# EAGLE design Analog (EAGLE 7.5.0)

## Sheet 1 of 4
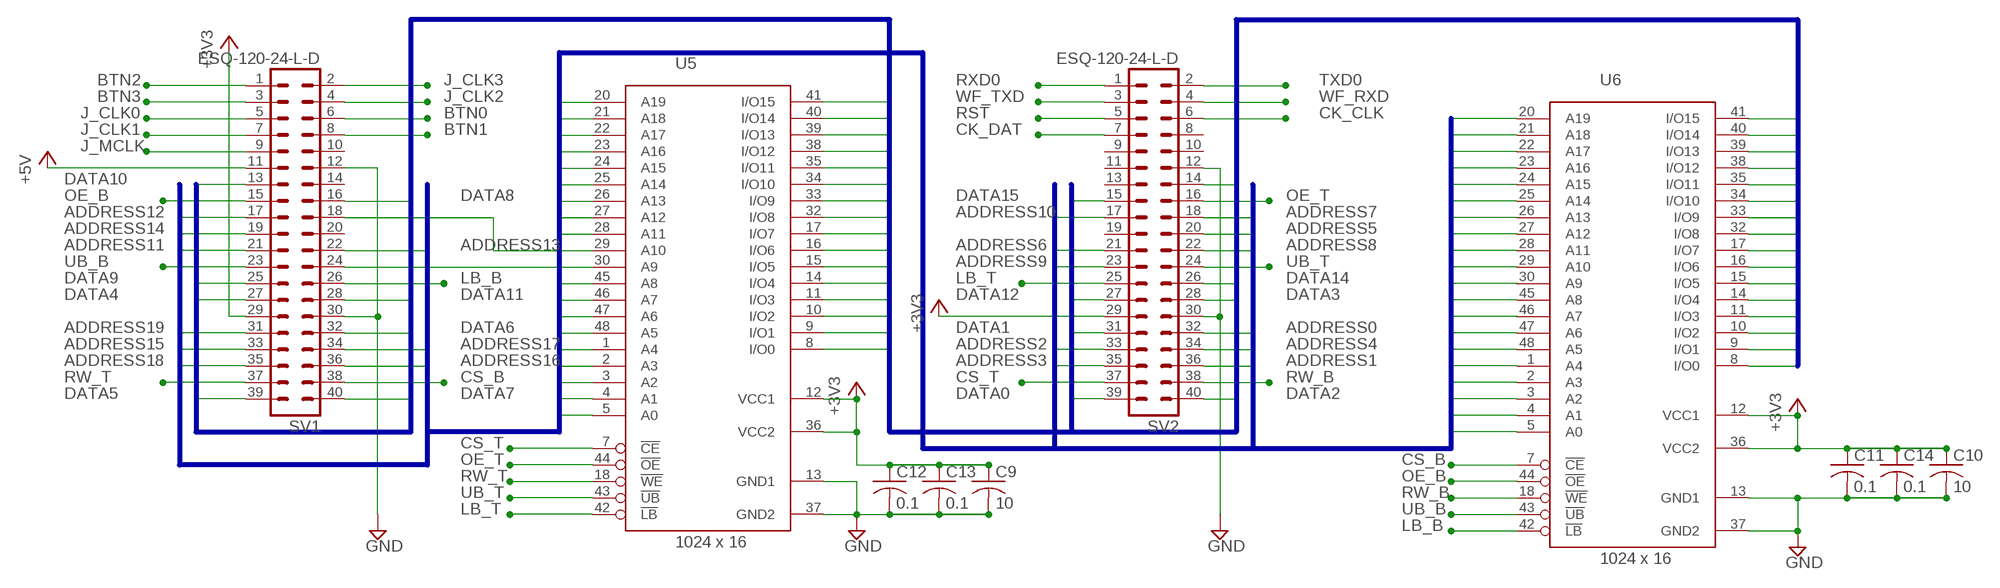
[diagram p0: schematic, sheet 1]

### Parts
C9  10  C-USC0805  [C0805]
C10  10  C-USC0805  [C0805]
C11  0.1  C-USC2012  [C2012]
C12  0.1  C-USC0805  [C0805]
C13  0.1  C-USC0805  [C0805]
C14  0.1  C-USC2012  [C2012]
SV1  ESQ-120-24-L-D  MA20-2  [MA20-2]
SV2  ESQ-120-24-L-D  MA20-2  [MA20-2]
U5  1024 x 16  IS62WV102416BLL-25T  [TSOP-I-48-12X40MM]
U6  1024 x 16  IS62WV102416BLL-25T  [TSOP-I-48-12X40MM]

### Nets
+3V3: C9.1 C10.1 C11.1 C12.1 C13.1 C14.1 SV1.29 SV2.29 U5.12(VCC1) U5.36(VCC2) U6.12(VCC1) U6.36(VCC2) ; also sheet 2,4
+5V: SV1.11 ; also sheet 3,4
ADDRESS0: SV2.32 U5.5(A0) U6.20(A19)
ADDRESS1: SV2.36 U5.4(A1) U6.21(A18)
ADDRESS2: SV2.33 U5.3(A2) U6.22(A17)
ADDRESS3: SV2.35 U5.2(A3) U6.23(A16)
ADDRESS4: SV2.34 U5.1(A4) U6.24(A15)
ADDRESS5: SV2.20 U5.48(A5) U6.25(A14)
ADDRESS6: SV2.21 U5.47(A6) U6.26(A13)
ADDRESS7: SV2.18 U5.46(A7) U6.27(A12)
ADDRESS8: SV2.22 U5.45(A8) U6.28(A11)
ADDRESS9: SV2.23 U6.30(A9)
ADDRESS9T: SV1.24 U5.30(A9)
ADDRESS10: SV2.17 U6.29(A10)
ADDRESS10T: SV1.18 U5.29(A10)
ADDRESS11: SV1.21 U5.28(A11) U6.45(A8)
ADDRESS12: SV1.17 U5.27(A12) U6.46(A7)
ADDRESS13: SV1.22 U5.26(A13) U6.47(A6)
ADDRESS14: SV1.19 U5.25(A14) U6.48(A5)
ADDRESS15: SV1.33 U5.24(A15) U6.1(A4)
ADDRESS16: SV1.36 U5.23(A16) U6.2(A3)
ADDRESS17: SV1.34 U5.22(A17) U6.3(A2)
ADDRESS18: SV1.35 U5.21(A18) U6.4(A1)
ADDRESS19: SV1.31 U5.20(A19) U6.5(A0)
BTN0: SV1.6 ; also sheet 3
BTN1: SV1.8 ; also sheet 3
BTN2: SV1.1 ; also sheet 3
BTN3: SV1.3 ; also sheet 3
CK_CLK: SV2.6 ; also sheet 4
CK_DAT: SV2.7 ; also sheet 4
CS_B: SV1.38 U6.7(!CE)
CS_T: SV2.37 U5.7(!CE)
DATA0: SV2.39 U5.8(I/O0) U6.17(I/O7)
DATA1: SV2.31 U5.9(I/O1) U6.16(I/O6)
DATA2: SV2.40 U5.10(I/O2) U6.15(I/O5)
DATA3: SV2.28 U5.11(I/O3) U6.14(I/O4)
DATA4: SV1.27 U5.14(I/O4) U6.11(I/O3)
DATA5: SV1.39 U5.15(I/O5) U6.10(I/O2)
DATA6: SV1.32 U5.16(I/O6) U6.9(I/O1)
DATA7: SV1.40 U5.17(I/O7) U6.8(I/O0)
DATA8: SV1.16 U5.32(I/O8) U6.41(I/O15)
DATA9: SV1.25 U5.33(I/O9) U6.40(I/O14)
DATA10: SV1.13 U5.34(I/O10) U6.39(I/O13)
DATA11: SV1.28 U5.35(I/O11) U6.38(I/O12)
DATA12: SV2.27 U5.38(I/O12) U6.35(I/O11)
DATA13: SV2.14 U5.39(I/O13) U6.34(I/O10)
DATA14: SV2.26 U5.40(I/O14) U6.33(I/O9)
DATA15: SV2.15 U5.41(I/O15) U6.32(I/O8)
GND: C9.2 C10.2 C11.2 C12.2 C13.2 C14.2 SV1.12 SV1.30 SV2.12 SV2.30 U5.13(GND1) U5.37(GND2) U6.13(GND1) U6.37(GND2) ; also sheet 2,3,4
J_CLK0: SV1.5 ; also sheet 3
J_CLK1: SV1.7 ; also sheet 3
J_CLK2: SV1.4 ; also sheet 3
J_CLK3: SV1.2 ; also sheet 3
J_MCLK: SV1.9 ; also sheet 3
LB_B: SV1.26 U6.42(!LB)
LB_T: SV2.25 U5.42(!LB)
OE_B: SV1.15 U6.44(!OE)
OE_T: SV2.16 U5.44(!OE)
RST: SV2.5 ; also sheet 4
RW_B: SV2.38 U6.18(!WE)
RW_T: SV1.37 U5.18(!WE)
RXD0: SV2.1 ; also sheet 2
TXD0: SV2.2 ; also sheet 2
UB_B: SV1.23 U6.43(!UB)
UB_T: SV2.24 U5.43(!UB)
WF_RXD: SV2.4 ; also sheet 4
WF_TXD: SV2.3 ; also sheet 4
Unconnected: SV1.10 SV1.14 SV1.20 SV2.8 SV2.9 SV2.10 SV2.11 SV2.13 SV2.19

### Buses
DATA[0..15]
ADDRESS[0..19]

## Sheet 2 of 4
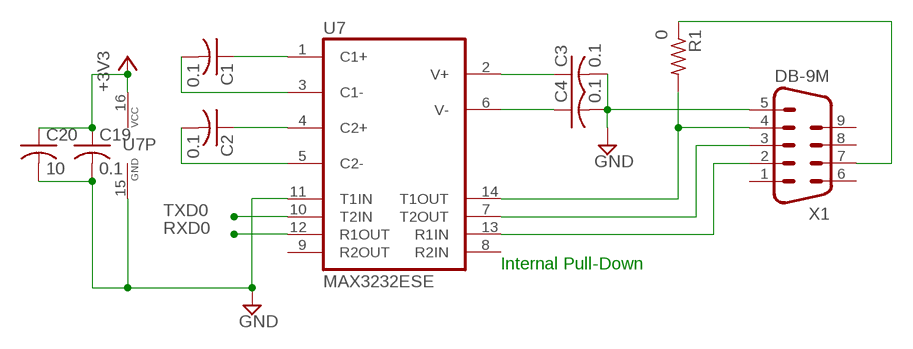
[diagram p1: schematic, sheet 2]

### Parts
C1  0.1  C-USC0805  [C0805]
C2  0.1  C-USC0805  [C0805]
C3  0.1  C-USC0805  [C0805]
C4  0.1  C-USC0805  [C0805]
C19  0.1  C-USC0805  [C0805]
C20  10  C-USC0805  [C0805]
R1  0  R-US_M0805  [M0805]
U7  MAX3232ESE  [SO16]
X1  DB-9M  M09HP  [M09HP]

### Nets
+3V3: C19.1 C20.1 U7.16(VCC) ; also sheet 1,4
GND: C3.2 C4.2 C19.2 C20.2 U7.11(T1IN) U7.15(GND) X1.5 ; also sheet 1,3,4
N$1: C1.1 U7.1(C1+)
N$2: C1.2 U7.3(C1-)
N$3: C2.1 U7.4(C2+)
N$4: C2.2 U7.5(C2-)
N$5: C3.1 U7.2(V+)
N$6: C4.1 U7.6(V-)
N$8: U7.13(R1IN) X1.2
N$9: U7.7(T2OUT) X1.3
N$27: R1.1 X1.7
N$28: R1.2 U7.14(T1OUT) X1.4
RXD0: U7.12(R1OUT) ; also sheet 1
TXD0: U7.10(T2IN) ; also sheet 1
Unconnected: U7.8(R2IN) U7.9(R2OUT) X1.1 X1.6 X1.8 X1.9

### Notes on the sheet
- Internal Pull-Down

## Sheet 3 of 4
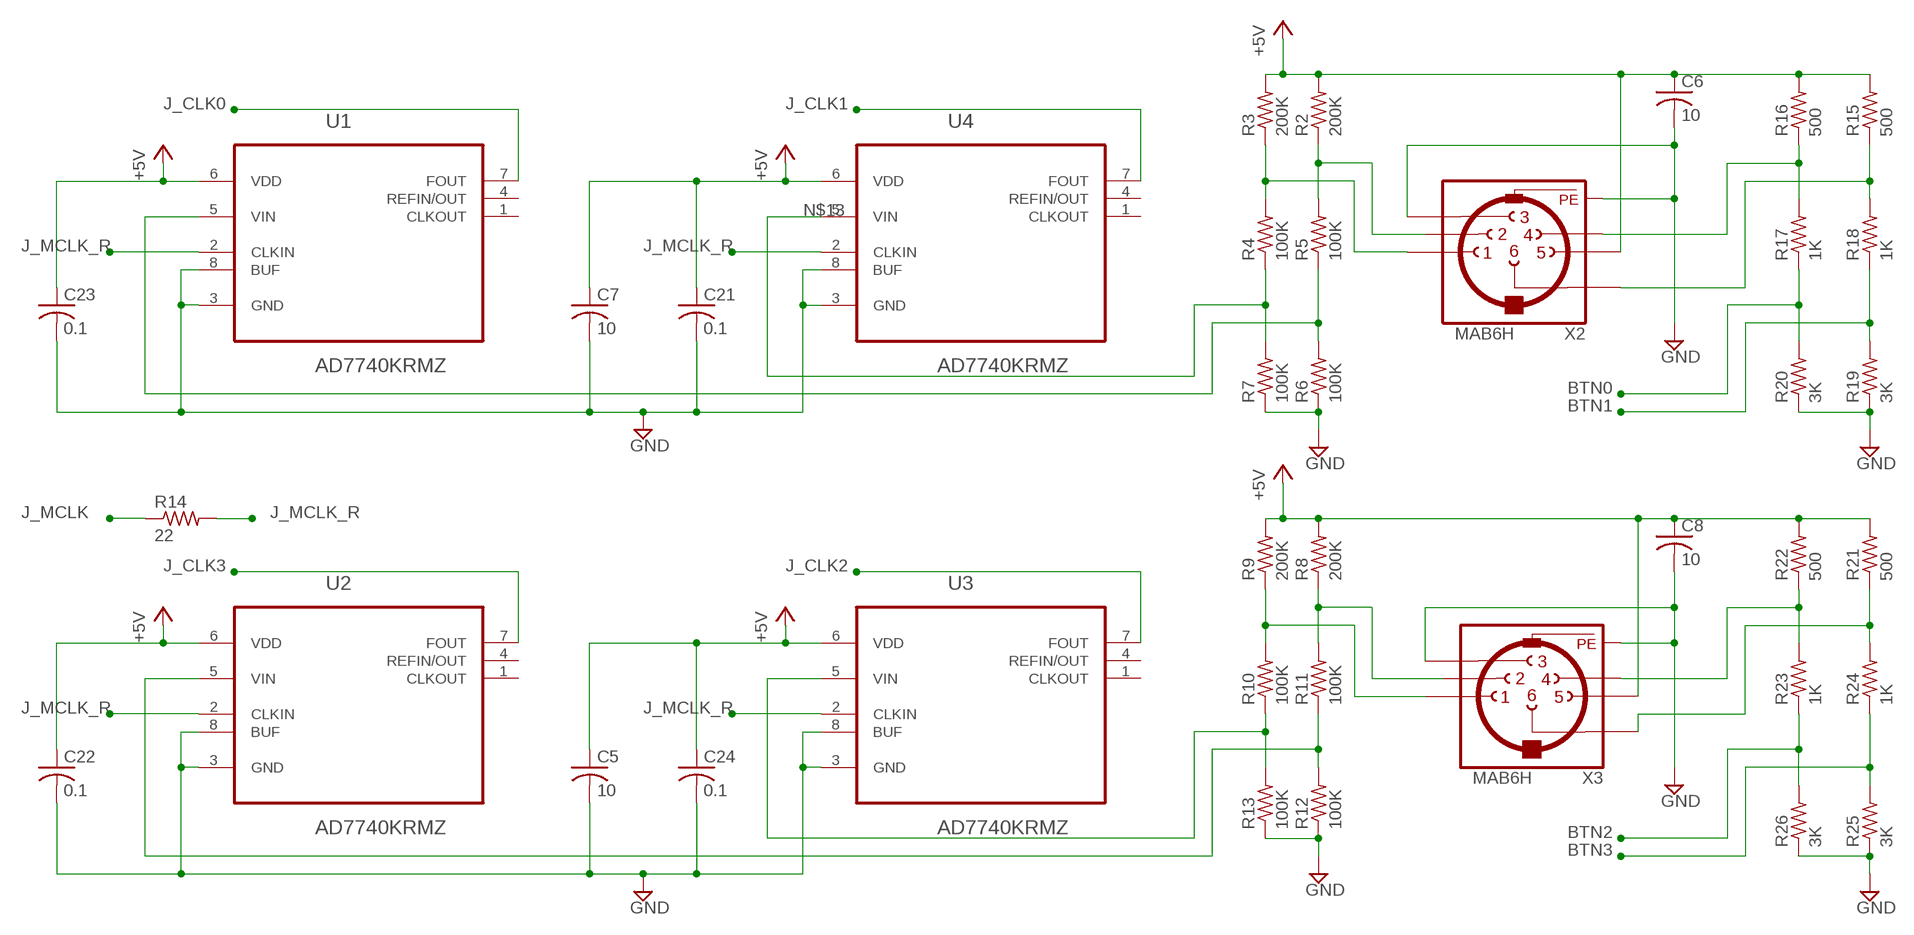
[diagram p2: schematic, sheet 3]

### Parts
C5  10  C-USC0805K  [C0805K]
C6  10  C-USC0805K  [C0805K]
C7  10  C-USC0805K  [C0805K]
C8  10  C-USC0805K  [C0805K]
C21  0.1  C-USC0805K  [C0805K]
C22  0.1  C-USC0805K  [C0805K]
C23  0.1  C-USC0805K  [C0805K]
C24  0.1  C-USC0805K  [C0805K]
R2  200K  R-US_M0805  [M0805]
R3  200K  R-US_M0805  [M0805]
R4  100K  R-US_M0805  [M0805]
R5  100K  R-US_M0805  [M0805]
R6  100K  R-US_M0805  [M0805]
R7  100K  R-US_M0805  [M0805]
R8  200K  R-US_M0805  [M0805]
R9  200K  R-US_M0805  [M0805]
R10  100K  R-US_M0805  [M0805]
R11  100K  R-US_M0805  [M0805]
R12  100K  R-US_M0805  [M0805]
R13  100K  R-US_M0805  [M0805]
R14  22  R-US_R0805  [R0805]
R15  500  R-US_R0805  [R0805]
R16  500  R-US_R0805  [R0805]
R17  1K  R-US_R0805  [R0805]
R18  1K  R-US_R0805  [R0805]
R19  3K  R-US_R0805  [R0805]
R20  3K  R-US_R0805  [R0805]
R21  500  R-US_R0805  [R0805]
R22  500  R-US_R0805  [R0805]
R23  1K  R-US_R0805  [R0805]
R24  1K  R-US_R0805  [R0805]
R25  3K  R-US_R0805  [R0805]
R26  3K  R-US_R0805  [R0805]
U1  AD7740KRMZ  [SOIC65P490X109-8N]
U2  AD7740KRMZ  [SOIC65P490X109-8N]
U3  AD7740KRMZ  [SOIC65P490X109-8N]
U4  AD7740KRMZ  [SOIC65P490X109-8N]
X2  MAB6H  [MAB6H]
X3  MAB6H  [MAB6H]

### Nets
+5V: C5.1 C6.1 C7.1 C8.1 C21.1 C22.1 C23.1 C24.1 R2.2 R3.2 R8.2 R9.2 R15.2 R16.2 R21.2 R22.2 U1.6(VDD) U2.6(VDD) U3.6(VDD) U4.6(VDD) X2.5 X3.5 ; also sheet 1,4
BTN0: R17.1 R20.2 ; also sheet 1
BTN1: R18.1 R19.2 ; also sheet 1
BTN2: R23.1 R26.2 ; also sheet 1
BTN3: R24.1 R25.2 ; also sheet 1
GND: C5.2 C6.2 C7.2 C8.2 C21.2 C22.2 C23.2 C24.2 R6.1 R7.1 R12.1 R13.1 R19.1 R20.1 R25.1 R26.1 U1.3(GND) U1.8(BUF) U2.3(GND) U2.8(BUF) U3.3(GND) U3.8(BUF) U4.3(GND) U4.8(BUF) X2.3 X2.PE X2.PE@(PE) X3.3 X3.PE X3.PE@(PE) ; also sheet 1,2,4
J_CLK0: U1.7(FOUT) ; also sheet 1
J_CLK1: U4.7(FOUT) ; also sheet 1
J_CLK2: U3.7(FOUT) ; also sheet 1
J_CLK3: U2.7(FOUT) ; also sheet 1
J_MCLK: R14.1 ; also sheet 1
J_MCLK_R: R14.2 U1.2(CLKIN) U2.2(CLKIN) U3.2(CLKIN) U4.2(CLKIN)
N$11: R22.1 R23.2 X3.4
N$12: R3.1 R4.2 X2.1
N$13: R4.1 R7.2 U4.5(VIN)
N$14: R5.1 R6.2 U1.5(VIN)
N$15: R2.1 R5.2 X2.2
N$16: R21.1 R24.2 X3.6
N$17: R9.1 R10.2 X3.1
N$18: R10.1 R13.2 U3.5(VIN)
N$19: R11.1 R12.2 U2.5(VIN)
N$20: R8.1 R11.2 X3.2
N$21: R16.1 R17.2 X2.4
N$22: R15.1 R18.2 X2.6
Unconnected: U1.1(CLKOUT) U1.4(REFIN/OUT) U2.1(CLKOUT) U2.4(REFIN/OUT) U3.1(CLKOUT) U3.4(REFIN/OUT) U4.1(CLKOUT) U4.4(REFIN/OUT)

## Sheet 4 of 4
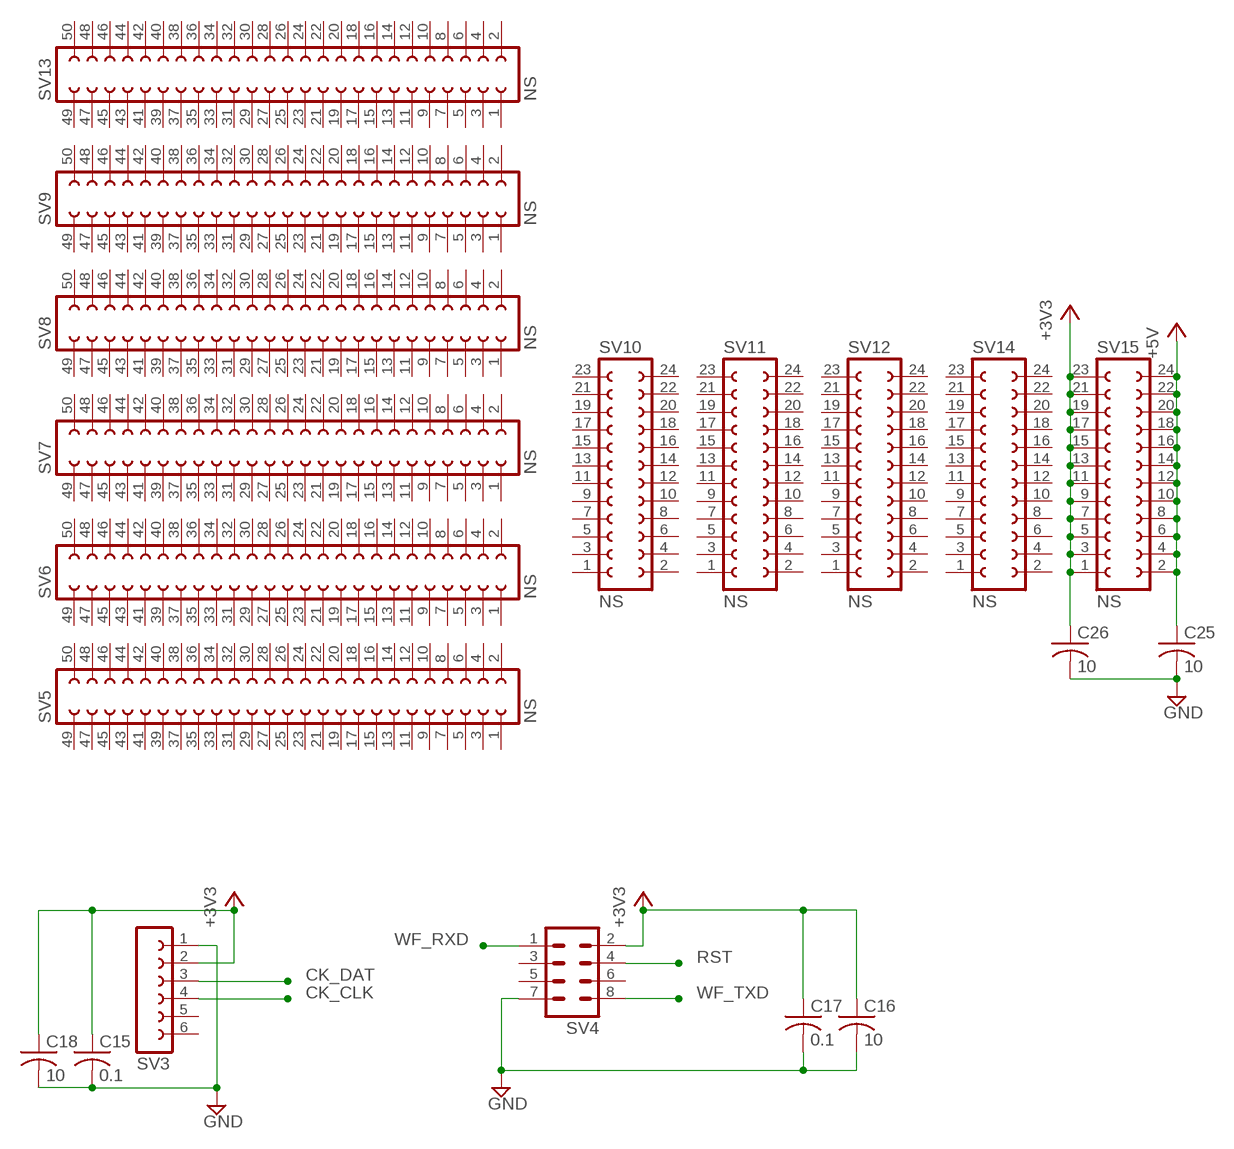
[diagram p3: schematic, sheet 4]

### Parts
C15  0.1  C-USC0805  [C0805]
C16  10  C-USC0805  [C0805]
C17  0.1  C-USC0805  [C0805]
C18  10  C-USC0805  [C0805]
C25  10  C-USC0805  [C0805]
C26  10  C-USC0805  [C0805]
SV3  FE06-1  [FE06]
SV4  MA04-2  [MA04-2]
SV5  NS  FE25-2  [FE25-2]
SV6  NS  FE25-2  [FE25-2]
SV7  NS  FE25-2  [FE25-2]
SV8  NS  FE25-2  [FE25-2]
SV9  NS  FE25-2  [FE25-2]
SV10  NS  FE12-2  [FE12-2]
SV11  NS  FE12-2  [FE12-2]
SV12  NS  FE12-2  [FE12-2]
SV13  NS  FE25-2  [FE25-2]
SV14  NS  FE12-2  [FE12-2]
SV15  NS  FE12-2  [FE12-2]

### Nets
+3V3: C15.1 C16.1 C17.1 C18.1 C26.1 SV3.2 SV4.2 SV15.1 SV15.3 SV15.5 SV15.7 SV15.9 SV15.11 SV15.13 SV15.15 SV15.17 SV15.19 SV15.21 SV15.23 ; also sheet 1,2
+5V: C25.1 SV15.2 SV15.4 SV15.6 SV15.8 SV15.10 SV15.12 SV15.14 SV15.16 SV15.18 SV15.20 SV15.22 SV15.24 ; also sheet 1,3
CK_CLK: SV3.4 ; also sheet 1
CK_DAT: SV3.3 ; also sheet 1
GND: C15.2 C16.2 C17.2 C18.2 C25.2 C26.2 SV3.1 SV4.7 ; also sheet 1,2,3
RST: SV4.4 ; also sheet 1
WF_RXD: SV4.1 ; also sheet 1
WF_TXD: SV4.8 ; also sheet 1
Unconnected: SV3.5 SV3.6 SV4.3 SV4.5 SV4.6 SV5.1 SV5.2 SV5.3 SV5.4 SV5.5 SV5.6 SV5.7 SV5.8 SV5.9 SV5.10 SV5.11 SV5.12 SV5.13 SV5.14 SV5.15 SV5.16 SV5.17 SV5.18 SV5.19 SV5.20 SV5.21 SV5.22 SV5.23 SV5.24 SV5.25 SV5.26 SV5.27 SV5.28 SV5.29 SV5.30 SV5.31 SV5.32 SV5.33 SV5.34 SV5.35 SV5.36 SV5.37 SV5.38 SV5.39 SV5.40 SV5.41 SV5.42 SV5.43 SV5.44 SV5.45 SV5.46 SV5.47 SV5.48 SV5.49 SV5.50 SV6.1 SV6.2 SV6.3 SV6.4 SV6.5 SV6.6 SV6.7 SV6.8 SV6.9 SV6.10 SV6.11 SV6.12 SV6.13 SV6.14 SV6.15 SV6.16 SV6.17 SV6.18 SV6.19 SV6.20 SV6.21 SV6.22 SV6.23 SV6.24 SV6.25 SV6.26 SV6.27 SV6.28 SV6.29 SV6.30 SV6.31 SV6.32 SV6.33 SV6.34 SV6.35 SV6.36 SV6.37 SV6.38 SV6.39 SV6.40 SV6.41 SV6.42 SV6.43 SV6.44 SV6.45 SV6.46 SV6.47 SV6.48 SV6.49 SV6.50 SV7.1 SV7.2 SV7.3 SV7.4 SV7.5 SV7.6 SV7.7 SV7.8 SV7.9 SV7.10 SV7.11 SV7.12 SV7.13 SV7.14 SV7.15 SV7.16 SV7.17 SV7.18 SV7.19 SV7.20 SV7.21 SV7.22 SV7.23 SV7.24 SV7.25 SV7.26 SV7.27 SV7.28 SV7.29 SV7.30 SV7.31 SV7.32 SV7.33 SV7.34 SV7.35 SV7.36 SV7.37 SV7.38 SV7.39 SV7.40 SV7.41 SV7.42 SV7.43 SV7.44 SV7.45 SV7.46 SV7.47 SV7.48 SV7.49 SV7.50 SV8.1 SV8.2 SV8.3 SV8.4 SV8.5 SV8.6 SV8.7 SV8.8 SV8.9 SV8.10 SV8.11 SV8.12 SV8.13 SV8.14 SV8.15 SV8.16 SV8.17 SV8.18 SV8.19 SV8.20 SV8.21 SV8.22 SV8.23 SV8.24 SV8.25 SV8.26 SV8.27 SV8.28 SV8.29 SV8.30 SV8.31 SV8.32 SV8.33 SV8.34 SV8.35 SV8.36 SV8.37 SV8.38 SV8.39 SV8.40 SV8.41 SV8.42 SV8.43 SV8.44 SV8.45 SV8.46 SV8.47 SV8.48 SV8.49 SV8.50 SV9.1 SV9.2 SV9.3 SV9.4 SV9.5 SV9.6 SV9.7 SV9.8 SV9.9 SV9.10 SV9.11 SV9.12 SV9.13 SV9.14 SV9.15 SV9.16 SV9.17 SV9.18 SV9.19 SV9.20 SV9.21 SV9.22 SV9.23 SV9.24 SV9.25 SV9.26 SV9.27 SV9.28 SV9.29 SV9.30 SV9.31 SV9.32 SV9.33 SV9.34 SV9.35 SV9.36 SV9.37 SV9.38 SV9.39 SV9.40 SV9.41 SV9.42 SV9.43 SV9.44 SV9.45 SV9.46 SV9.47 SV9.48 SV9.49 SV9.50 SV10.1 SV10.2 SV10.3 SV10.4 SV10.5 SV10.6 SV10.7 SV10.8 SV10.9 SV10.10 SV10.11 SV10.12 SV10.13 SV10.14 SV10.15 SV10.16 SV10.17 SV10.18 SV10.19 SV10.20 SV10.21 SV10.22 SV10.23 SV10.24 SV11.1 SV11.2 SV11.3 SV11.4 SV11.5 SV11.6 SV11.7 SV11.8 SV11.9 SV11.10 SV11.11 SV11.12 SV11.13 SV11.14 SV11.15 SV11.16 SV11.17 SV11.18 SV11.19 SV11.20 SV11.21 SV11.22 SV11.23 SV11.24 SV12.1 SV12.2 SV12.3 SV12.4 SV12.5 SV12.6 SV12.7 SV12.8 SV12.9 SV12.10 SV12.11 SV12.12 SV12.13 SV12.14 SV12.15 SV12.16 SV12.17 SV12.18 SV12.19 SV12.20 SV12.21 SV12.22 SV12.23 SV12.24 SV13.1 SV13.2 SV13.3 SV13.4 SV13.5 SV13.6 SV13.7 SV13.8 SV13.9 SV13.10 SV13.11 SV13.12 SV13.13 SV13.14 SV13.15 SV13.16 SV13.17 SV13.18 SV13.19 SV13.20 SV13.21 SV13.22 SV13.23 SV13.24 SV13.25 SV13.26 SV13.27 SV13.28 SV13.29 SV13.30 SV13.31 SV13.32 SV13.33 SV13.34 SV13.35 SV13.36 SV13.37 SV13.38 SV13.39 SV13.40 SV13.41 SV13.42 SV13.43 SV13.44 SV13.45 SV13.46 SV13.47 SV13.48 SV13.49 SV13.50 SV14.1 SV14.2 SV14.3 SV14.4 SV14.5 SV14.6 SV14.7 SV14.8 SV14.9 SV14.10 SV14.11 SV14.12 SV14.13 SV14.14 SV14.15 SV14.16 SV14.17 SV14.18 SV14.19 SV14.20 SV14.21 SV14.22 SV14.23 SV14.24

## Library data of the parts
C1-C26 = rcl:C-US: CAPACITOR, American symbol
R1-R26 = rcl:R-US_: RESISTOR, American symbol
SV1 SV2 = con-lstb:MA20-2: PIN HEADER; OC_FARNELL: unknown; OC_NEWARK: unknown
SV3 = con-lsta:FE06-1: FEMALE HEADER; OC_FARNELL: unknown; OC_NEWARK: unknown
SV4 = con-lstb:MA04-2: PIN HEADER; OC_FARNELL: unknown; OC_NEWARK: unknown
SV5-SV9 SV13 = Gary_LBR:FE25-2: FEMALE HEADER; OC_FARNELL: unknown; OC_NEWARK: unknown
SV10-SV12 SV14 SV15 = Gary_LBR:FE12-2: FEMALE HEADER; OC_FARNELL: unknown; OC_NEWARK: unknown
U1-U4 = Analog Devices_By_element14_Batch_1:AD7740KRMZ: 3 V/5 V Low Power, Synchronous Voltage-to-Frequency Converter; MPN: AD7740KRMZ; OC_FARNELL: 1661051; OC_NEWARK: 59K5406; PACKAGE: SOIC-8; SUPPLIER: Analog Devices
U5 U6 = Gary_LBR:IS62WV102416BLL-*: 1024k x 16 high- speed low power CMOS static RAM 25ns access time 3.6V power supply
U7 = maxim:MAX3232*: True RS-232 Transceivers 3.0V to 5.5V, Low-Power up to 1Mbps, Using Four 0.1µF External Capacitors Source: http://pdfserv.maxim-ic.com/en/ds/MAX3222-MAX3241.pdf; MF: MAXIM; MPN: MAX3232ESE; OC_FARNELL: 9725539; OC_NEWARK: 79C3880
X1 = con-subd:M09: SUB-D; OC_FARNELL: unknown; OC_NEWARK: unknown
X2 X3 = con-hirschmann:MAB6H: Female CONNECTOR 6 pins with shield, horizontal (DIN 45322); MF: FARNELL; MPN: MAB 6 H; OC_FARNELL: 809901; OC_NEWARK: 67C7887

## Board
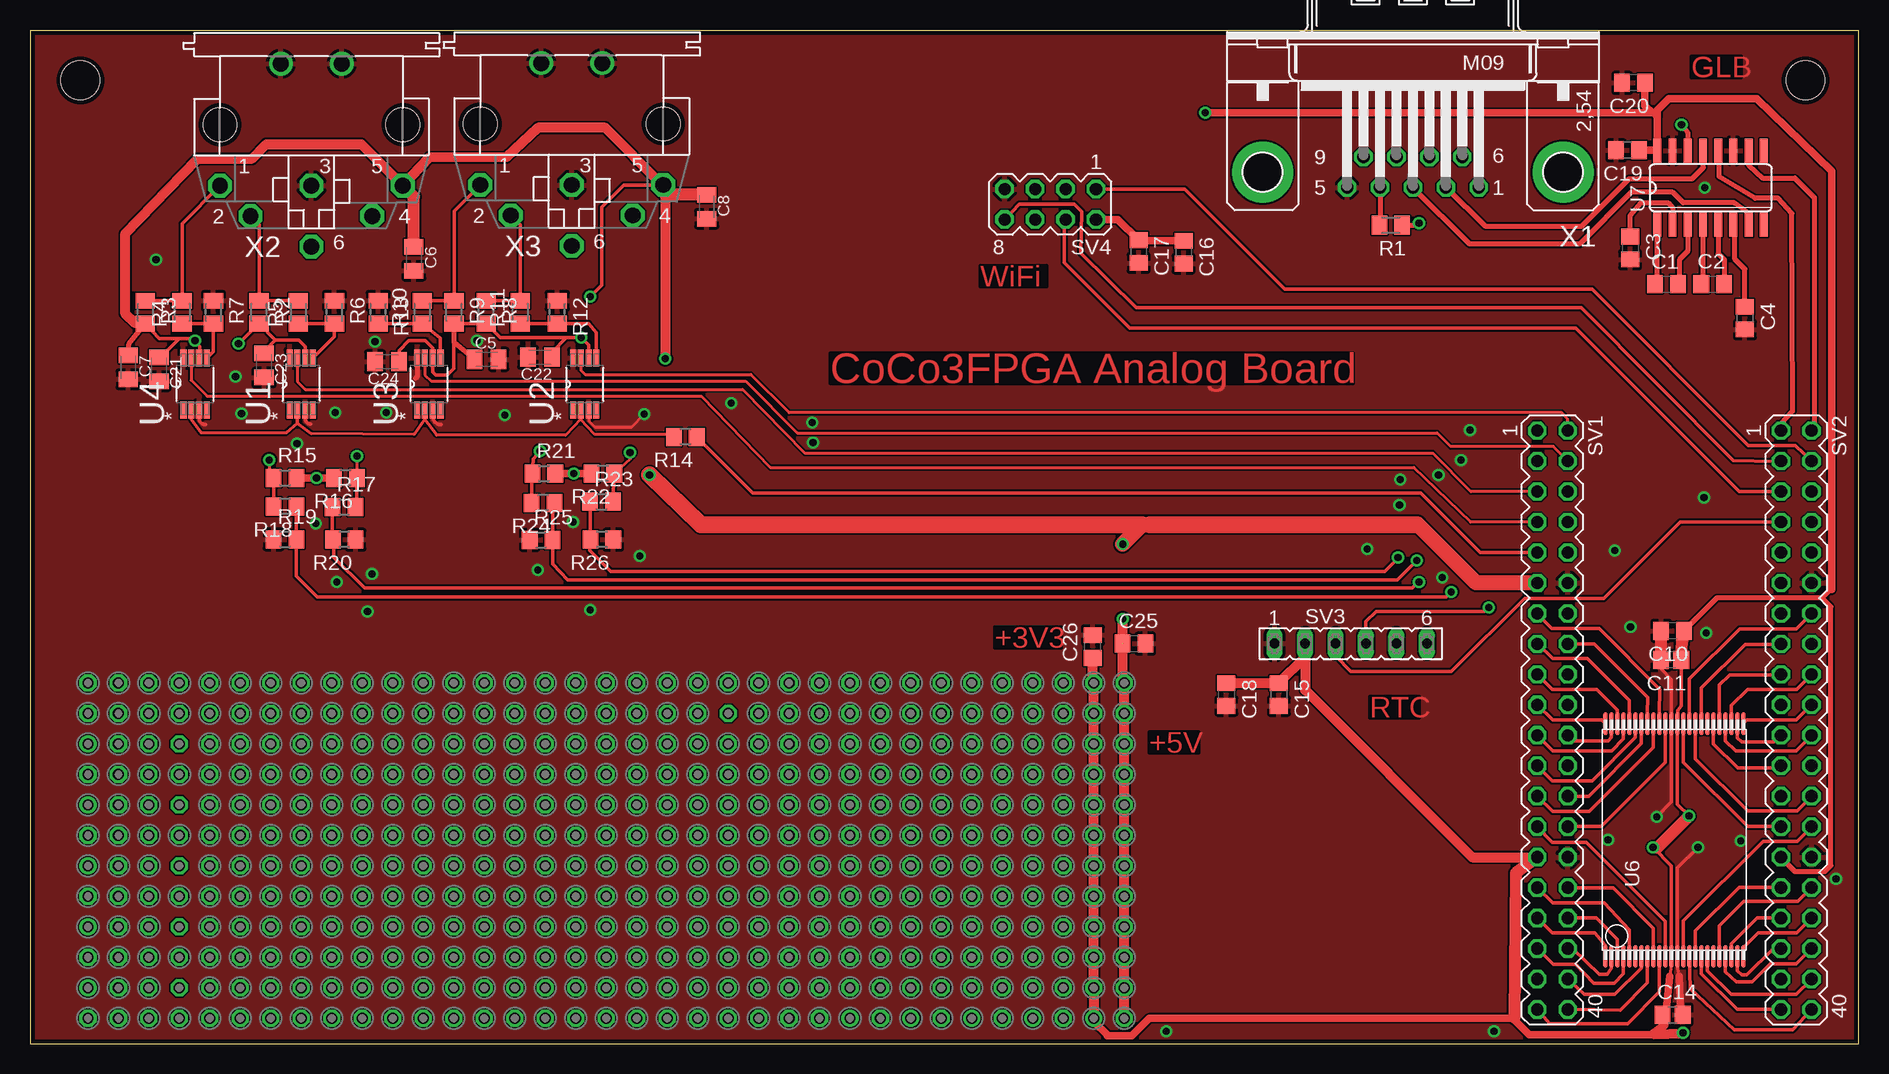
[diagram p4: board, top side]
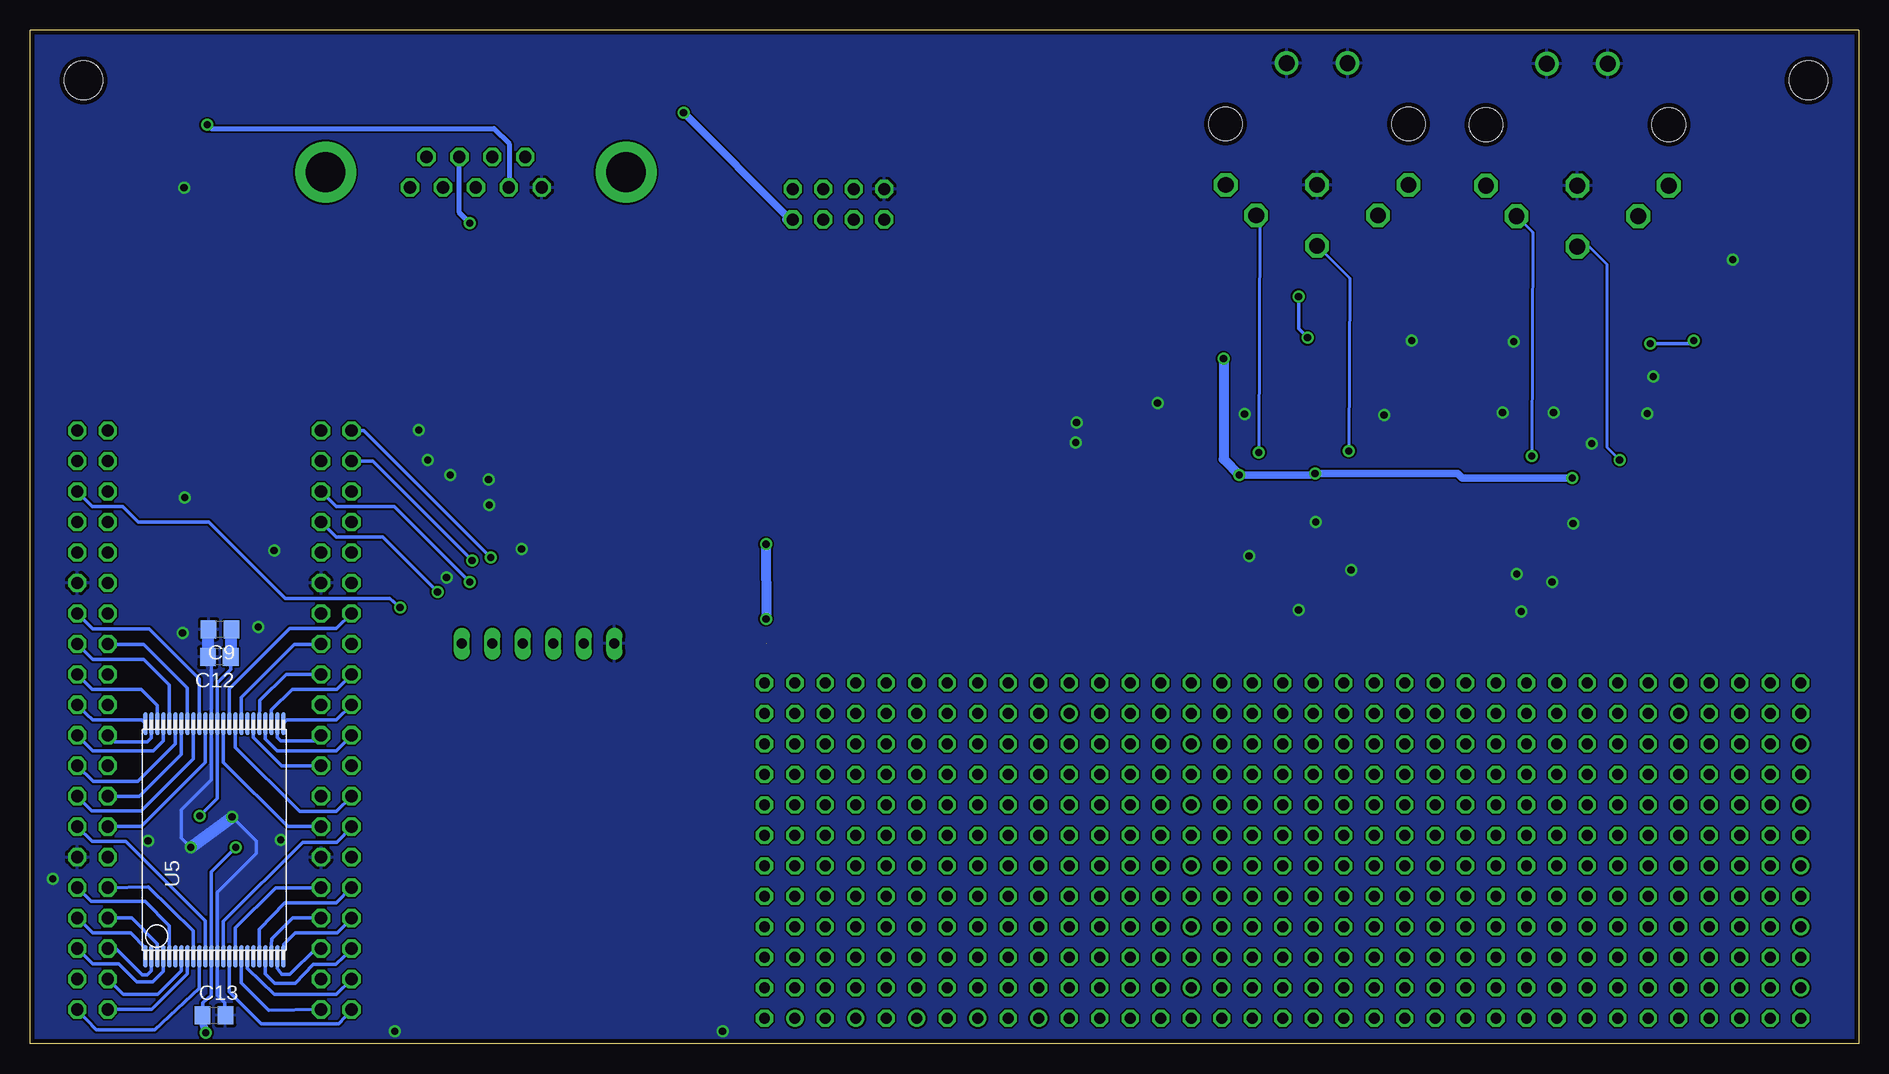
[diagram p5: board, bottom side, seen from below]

Size 152.4 x 84.53 mm. Coordinates in mm from the lower left corner, seen from the top.
Outline: 0,0 152.4,0 152.4,84.53 0,84.53 0,0
Copper layers (1*16): Top 0.035559375mm / dielectric 1.501140625mm / Bottom 0.035559375mm
Design rules "typical_4pcb": minimum track width 10mil, minimum drill 15mil, track to track 6mil, track to pad 6mil, pad to pad 6mil, via to via 6mil, smd to smd 6mil, copper to edge 15mil, drill to drill 8mil, minimum pad ring 10mil, minimum via ring 8mil, stop-mask expansion 4mil, vias tented up to drill 0mil, thermal gap 10mil
Holes 3.2 mm at 147.96,80.34 4.19,80.34

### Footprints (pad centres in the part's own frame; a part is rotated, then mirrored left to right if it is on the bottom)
C0805 = smd 1.3 x 1.5: 1 -0.95,0; 2 0.95,0
C0805K = smd 1.3 x 1.6: 1 -1,0; 2 1,0
C2012 = smd 1.3 x 1.5: 1 -0.85,0; 2 0.85,0
M0805 = smd 1.3 x 1.6: 1 -0.95,0; 2 0.95,0
R0805 = smd 1.3 x 1.5: 1 -0.95,0; 2 0.95,0
MA20-2 = drill 1.016 octagon: 1 -24.13,-1.27; 2 -24.13,1.27; 3 -21.59,-1.27; 4 -21.59,1.27; 5 -19.05,-1.27; 6 -19.05,1.27; 7 -16.51,-1.27; 8 -16.51,1.27; 9 -13.97,-1.27; 10 -13.97,1.27; 11 -11.43,-1.27; 12 -11.43,1.27; 13 -8.89,-1.27; 14 -8.89,1.27; 15 -6.35,-1.27; 16 -6.35,1.27; 17 -3.81,-1.27; 18 -3.81,1.27; 19 -1.27,-1.27; 20 -1.27,1.27; 21 1.27,-1.27; 22 1.27,1.27; 23 3.81,-1.27; 24 3.81,1.27; 25 6.35,-1.27; 26 6.35,1.27; 27 8.89,-1.27; 28 8.89,1.27; 29 11.43,-1.27; 30 11.43,1.27; 31 13.97,-1.27; 32 13.97,1.27; 33 16.51,-1.27; 34 16.51,1.27; 35 19.05,-1.27; 36 19.05,1.27; 37 21.59,-1.27; 38 21.59,1.27; 39 24.13,-1.27; 40 24.13,1.27
FE06 = drill 0.813 long: 1 -6.35,0; 2 -3.81,0; 3 -1.27,0; 4 1.27,0; 5 3.81,0; 6 6.35,0
MA04-2 = drill 1.016 octagon: 1 -3.81,-1.27; 2 -3.81,1.27; 3 -1.27,-1.27; 4 -1.27,1.27; 5 1.27,-1.27; 6 1.27,1.27; 7 3.81,-1.27; 8 3.81,1.27
FE25-2 = drill 0.914: 1 -30.48,1.27; 41 20.32,1.27 | drill 0.914 octagon: 2 -30.48,-1.27; 3 -27.94,1.27; 4 -27.94,-1.27; 5 -25.4,1.27; 6 -25.4,-1.27; 7 -22.86,1.27; 8 -22.86,-1.27; 9 -20.32,1.27; 10 -20.32,-1.27; 11 -17.78,1.27; 12 -17.78,-1.27; 13 -15.24,1.27; 14 -15.24,-1.27; 15 -12.7,1.27; 16 -12.7,-1.27; 17 -10.16,1.27; 18 -10.16,-1.27; 19 -7.62,1.27; 20 -7.62,-1.27; 21 -5.08,1.27; 22 -5.08,-1.27; 23 -2.54,1.27; 24 -2.54,-1.27; 25 0,1.27; 26 0,-1.27; 27 2.54,1.27; 28 2.54,-1.27; 29 5.08,1.27; 30 5.08,-1.27; 31 7.62,1.27; 32 7.62,-1.27; 33 10.16,1.27; 34 10.16,-1.27; 35 12.7,1.27; 36 12.7,-1.27; 37 15.24,1.27; 38 15.24,-1.27; 39 17.78,1.27; 40 17.78,-1.27; 42 20.32,-1.27; 43 22.86,1.27; 44 22.86,-1.27; 45 25.4,1.27; 46 25.4,-1.27; 47 27.94,1.27; 48 27.94,-1.27; 49 30.48,1.27; 50 30.48,-1.27
FE12-2 = drill 0.914: 1 -13.97,1.27 | drill 0.914 octagon: 2 -13.97,-1.27; 3 -11.43,1.27; 4 -11.43,-1.27; 5 -8.89,1.27; 6 -8.89,-1.27; 7 -6.35,1.27; 8 -6.35,-1.27; 9 -3.81,1.27; 10 -3.81,-1.27; 11 -1.27,1.27; 12 -1.27,-1.27; 13 1.27,1.27; 14 1.27,-1.27; 15 3.81,1.27; 16 3.81,-1.27; 17 6.35,1.27; 18 6.35,-1.27; 19 8.89,1.27; 20 8.89,-1.27; 21 11.43,1.27; 22 11.43,-1.27; 23 13.97,1.27; 24 13.97,-1.27
SOIC65P490X109-8N = smd 1.422 x 0.508: 1 -2.159,0.965; 2 -2.159,0.33; 3 -2.159,-0.33; 4 -2.159,-0.965; 5 2.159,-0.965; 6 2.159,-0.33; 7 2.159,0.33; 8 2.159,0.965
TSOP-I-48-12X40MM = smd 1.9 x 0.34: 1 -9.7,5.75; 2 -9.7,5.25; 3 -9.7,4.75; 4 -9.7,4.25; 5 -9.7,3.75; 6 -9.7,3.25; 7 -9.7,2.75; 8 -9.7,2.25; 9 -9.7,1.75; 10 -9.7,1.25; 11 -9.7,0.75; 12 -9.7,0.25; 13 -9.7,-0.25; 14 -9.7,-0.75; 15 -9.7,-1.25; 16 -9.7,-1.75; 17 -9.7,-2.25; 18 -9.7,-2.75; 19 -9.7,-3.25; 20 -9.7,-3.75; 21 -9.7,-4.25; 22 -9.7,-4.75; 23 -9.7,-5.25; 24 -9.7,-5.75; 25 9.7,-5.75; 26 9.7,-5.25; 27 9.7,-4.75; 28 9.7,-4.25; 29 9.7,-3.75; 30 9.7,-3.25; 31 9.7,-2.75; 32 9.7,-2.25; 33 9.7,-1.75; 34 9.7,-1.25; 35 9.7,-0.75; 36 9.7,-0.25; 37 9.7,0.25; 38 9.7,0.75; 39 9.7,1.25; 40 9.7,1.75; 41 9.7,2.25; 42 9.7,2.75; 43 9.7,3.25; 44 9.7,3.75; 45 9.7,4.25; 46 9.7,4.75; 47 9.7,5.25; 48 9.7,5.75
SO16 = smd 0.66 x 2.032: 1 -4.445,-3.073; 2 -3.175,-3.073; 3 -1.905,-3.073; 4 -0.635,-3.073; 5 0.635,-3.073; 6 1.905,-3.073; 7 3.175,-3.073; 8 4.445,-3.073; 9 4.445,3.073; 10 3.175,3.073; 11 1.905,3.073; 12 0.635,3.073; 13 -0.635,3.073; 14 -1.905,3.073; 15 -3.175,3.073; 16 -4.445,3.073
M09HP = drill 1.016 octagon: 1 -5.486,1.27; 2 -2.743,1.27; 3 0,1.27; 4 2.743,1.27; 5 5.486,1.27; 6 -4.115,-1.27; 7 -1.372,-1.27; 8 1.372,-1.27; 9 4.115,-1.27 | drill 3.302 pad 5.08: G1 -12.522,0; G2 12.522,0
MAB6H = drill 1.321 octagon: 1 7.62,5.08; 2 5.08,7.62; 3 0,5.08; 4 -5.08,7.62; 5 -7.62,5.08; 6 0,10.16 | drill 1.321: PE -2.54,-5.08; PE@ 2.54,-5.08 | hole 2.794: 7.62,0; -7.62,0

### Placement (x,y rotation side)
C1  136.37,63.34 0 top
C2  140.22,63.35 0 top
C3  133.35,66.35 270 top
C4  142.91,60.51 270 top
C5  38.06,57.07 0 top
C6  31.99,65.46 270 top
C7  8.19,56.41 270 top
C8  56.4,69.8 270 top
C9  136.56,34.56 180 bottom
C10  136.88,34.44 180 top
C11  136.75,32 180 top
C12  136.62,32.25 180 bottom
C13  137.06,2.38 0 bottom
C14  136.88,2.44 0 top
C15  104.06,29.12 270 top
C16  96.12,66 270 top
C17  92.38,66.06 270 top
C18  99.69,29.12 270 top
C19  133.12,74.5 180 top
C20  133.62,80.12 180 top
C21  10.75,56.25 270 top
C22  42.5,57.25 180 top
C23  19.5,56.56 270 top
C24  29.75,56.88 180 top
C25  92,33.38 0 top
C26  88.56,33.12 90 top
R1  113.39,68.25 180 top
R2  19.09,61 270 top
R3  9.62,61 270 top
R4  12.67,61 90 top
R5  22.35,61 90 top
R6  25.37,61 270 top
R7  15.29,61 270 top
R8  38.02,61 270 top
R9  35.34,61 270 top
R10  32.67,61 90 top
R11  40.84,61 90 top
R12  43.94,61 270 top
R13  29.01,61 270 top
R14  54.61,50.61 180 top
R15  21.24,47.19 0 top
R16  26.3,47.19 180 top
R17  26.17,44.77 0 top
R18  21.25,44.8 180 top
R19  21.25,42.07 0 top
R20  26.19,42.04 180 top
R21  42.82,47.56 0 top
R22  47.74,47.56 180 top
R23  47.63,45.2 0 top
R24  42.76,45.11 180 top
R25  42.59,42.02 0 top
R26  47.65,42.04 180 top
SV1  126.87,27 270 top
SV2  147.19,27 270 top
SV3  110.06,33.38 0 top
SV4  85.03,70 180 top
SV5  35.31,28.81 180 top
SV6  35.31,23.73 0 top
SV7  35.31,18.65 0 top
SV8  35.31,13.57 0 top
SV9  35.31,8.49 0 top
SV10  69.6,16.11 90 top
SV11  74.68,16.11 90 top
SV12  79.76,16.11 90 top
SV13  35.31,3.41 0 top
SV14  84.84,16.11 90 top
SV15  89.92,16.11 90 top
U1  22.6,55 90 top
U2  46.23,55 90 top
U3  33.24,55 90 top
U4  13.76,55 90 top
U5  137.03,17 90 bottom
U6  137.03,17 90 top
U7  140.05,71.38 0 top
X1  115.25,72.67 180 top
X2  23.45,76.63 180 top
X3  45.15,76.69 180 top

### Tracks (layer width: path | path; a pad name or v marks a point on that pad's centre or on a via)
+3V3  (via drill 0.6)
  Top 0.254: 137.31,27.55 U6.36 | 136.62,5.62 136.75,6.25 U6.12 | 123.56,2.12 123.62,2.12 123.69,2.12 123.69,2.19
  Top 0.305: C11.1 137.6,28.16 137.31,27.81 137.31,27.55 | v138.25,19 137.28,19.97 U6.36 | U6.12 136.78,14.84 v135.25,16.38
  Top 0.406: C14.1 136.12,2.44 136.31,2.44 | SV2.29 145.92,15.51 147.06,14.38 149.56,14.38 150.06,14.88 150.06,36.44 149.31,37.19 | 149.31,37.19 140.57,37.19 C10.1 | 150.12,37.88 150,37.88 149.31,37.19
  Top 0.61: SV4.2 90.66,68.73 C17.1 92.44,66.95 C16.1 | 136.31,2.44 136.62,5.62 | 135.06,0.75 136.12,1.56 | 135.06,0.75 135.31,0.81 | 150.12,37.88 150.12,72.75 143.88,78.81 136.56,78.81 135.6,77.86 135.6,77.31 | 135.6,77.31 U7.16 135.56,74.5 C19.1 | v97.94,77.62 135.19,77.62 | 135.19,77.62 135.29,77.62 135.6,77.31 | C20.1 134.57,78.24 135.19,77.62 | 135.06,0.75 124.94,0.75 123.56,2.12 | SV15.1 88.65,1.85 89.75,0.75 89.75,0.69 91.81,0.69 93.25,2.12 123.62,2.12
  Top 0.813: 136.12,1.56 136.12,2.44 | 135.31,0.81 137.81,0.88 | SV1.29 120.18,15.57 106.25,29.5 SV3.2 106.25,32.27 C15.1 C18.1 | SV15.1 SV15.3 SV15.5 SV15.7 SV15.9 SV15.11 SV15.13 SV15.15 SV15.17 SV15.19 SV15.21 SV15.23 88.58,30.16 C26.1
  Top 1.016: C11.1 arc-10 C10.1 | SV1.29 123.81,14.25 123.69,2.19 | v135.25,16.38 135.62,16.38 v138.25,19
  Bottom 0.305: v138.25,19 136.78,20.47 U5.36 136.78,30.09 135.68,31.2 C12.1 | v135.25,16.38 137.28,14.34 U5.12 137.28,6.43 137.31,4.06 138.01,3.42 C13.1
  Bottom 0.61: C13.1 138.01,1.76 137.93,1.51 v137.75,0.94 | 89.42,68.73 SV4.2 89.04,68.73 v97.94,77.62
  Bottom 0.813: C9.1 135.68,34.5
  Bottom 1.016: 135.68,34.5 C12.1
+5V  (via drill 0.6)  (1 unrouted)
  Top 0.305: R3.2 10.79,58.81 12.44,58.81 | U1.6 22.93,58.13 22.38,58.69 20.45,58.69 | 20.45,58.69 R2.2 19.05,60.05 v17.38,58.38 | U2.6 46.56,58.25 v45.94,58.88 44.69,58.88 | 44.69,58.88 39.2,58.88 R8.2 R9.2 35.31,60.02 35.31,56.31 34.75,55.75 33.81,55.75 33.56,56 33.56,56.06 33.57,56.07 U3.6 33.56,58 32.94,58.62 31.56,58.62 30.75,57.81 C24.1 | U4.6 14.12,57.2 14.12,58.12 v13.75,58.62 13.56,58.81 12.44,58.81 | X3.5 49.49,71.61 47.62,69.75 47.62,63.25 v46.69,62.31 | C21.1 10.88,57.25 12.44,58.81 | C23.1 19.5,57.73 20.45,58.69 | C22.1 43.5,57.69 44.69,58.88
  Top 0.406: C5.1 35.34,58.47 R9.2 | C7.1 8.24,58.34 R3.2
  Top 0.61: R21.2 v45.31,47.56 R22.2 | R16.2 v23.88,47.19 R15.2 | R3.2 8.76,60.11
  Top 0.813: v52.94,57.12 52.95,70.42 X3.5 52.7,71.61 47.94,76.38 42.31,76.38 39.69,73.94 33.27,73.88 X2.5 27.62,75 19.69,75 18.5,73.81 13.94,73.75 7.94,67.56 7.94,60.88 8.76,60.11 | 91.06,33.39 v91.06,35.44 | 91.19,33.23 C25.1 91.05,30.23 SV15.24 SV15.22 SV15.20 SV15.18 SV15.16 SV15.14 SV15.12 SV15.10 SV15.8 SV15.6 SV15.4 SV15.2
  Top 1.016: C6.1 31.99,70.63 X2.5 | C8.1 53.58,70.8 X3.5
  Top 1.27: SV1.11 120.51,38.43 115.62,43.31 115.6,43.29 | 55.88,43.31 55.9,43.29 | v91.06,41.66 92.69,43.29 93.31,43.29
  Top 1.422: 55.88,43.31 v51.62,47.44 | 55.9,43.29 92.69,43.29 | 93.31,43.29 115.6,43.29
  Bottom 0.305: v17.38,58.38 13.94,58.38 v13.75,58.62 | v46.69,62.31 46.69,59.62 v45.94,58.88
  Bottom 0.61: v51.62,47.44 45.44,47.44 v45.31,47.56 33.44,47.56 33.06,47.19 v23.88,47.19
  Bottom 0.813: v52.94,57.12 52.94,48.75 v51.62,47.44 | v91.06,35.44 91,35.5 v91.06,41.66
ADDRESS0
  Top 0.305: U6.20 140.78,9.85 142.81,11.88 147.31,11.88 SV2.32
  Bottom 0.305: SV2.32 147.31,11.88 142.81,11.88 140.78,9.84 140.78,8.15 U6.20
ADDRESS1
  Top 0.305: U6.21 141.28,6.03 142.19,5.19 143.5,5.19 145,6.69 147.2,6.69 SV2.36
  Bottom 0.305: SV2.36 147.19,6.69 145,6.69 143.5,5.19 142.19,5.19 141.28,6.03 141.28,6.06 141.28,7.27 U6.21
ADDRESS2
  Top 0.305: U6.22 141.78,8.35 143.94,10.5 SV2.33
  Bottom 0.305: SV2.33 143.93,10.49 141.78,8.34 U6.22
ADDRESS3
  Top 0.305: U6.23 142.28,6.09 142.62,5.75 143.06,5.75 145.25,7.94 145.91,7.94 SV2.35
  Bottom 0.305: SV2.35 145.26,7.95 143.06,5.75 142.62,5.75 142.28,6.09 142.28,7.24 U6.23
ADDRESS4
  Top 0.305: U6.24 142.8,8.05 144,9.25 147.22,9.25 SV2.34
  Bottom 0.305: SV2.34 148.43,10.49 147.19,9.25 144,9.25 142.81,8 142.81,7.27 U6.24
ADDRESS5
  Top 0.305: SV2.20 147.19,27 143.08,27 U6.25
  Bottom 0.305: U6.25 143.08,27 147.19,27 148.21,27.96 SV2.20
ADDRESS6
  Top 0.305: U6.26 142.28,25.53 142.62,25.19 145.32,25.19 SV2.21
  Bottom 0.305: U6.26 142.28,25.53 142.62,25.19 145.32,25.19 SV2.21
ADDRESS7
  Top 0.305: U6.27 141.78,28.22 143.12,29.56 147.22,29.56 SV2.18
  Bottom 0.305: U6.27 141.78,28.22 143.12,29.56 147.22,29.56 SV2.18
ADDRESS8
  Top 0.305: U6.28 141.28,25.28 142.12,24.44 147.17,24.44 SV2.22
  Bottom 0.305: U6.28 141.28,25.28 142.12,24.44 147.17,24.44 SV2.22
ADDRESS9
  Top 0.305: U6.30 140.28,25.03 142.31,23 145.73,23 SV2.23
ADDRESS9T
  Bottom 0.305: U5.30 133.78,25.53 131.44,23.19 128.27,23.19 SV1.24
ADDRESS10
  Top 0.305: U6.29 140.78,29.91 141.62,30.75 145.86,30.75 SV2.17
ADDRESS10T
  Bottom 0.305: U5.29 133.25,28.65 131.06,30.81 SV1.18
ADDRESS11
  Top 0.305: SV1.21 125.73,25.58 126.88,24.44 131.81,24.44 132.78,25.41 U6.45
  Bottom 0.305: U6.45 132.78,25.41 131.81,24.44 126.89,24.44 SV1.21
ADDRESS12
  Top 0.305: U6.46 132.28,27.84 130.56,29.56 126.85,29.56 SV1.17
  Bottom 0.305: U6.46 132.28,27.84 130.56,29.56 126.85,29.56 SV1.17
ADDRESS13
  Top 0.305: U6.47 131.78,25.53 131.5,25.25 128.62,25.25 SV1.22
  Bottom 0.305: U6.47 131.78,25.53 131.5,25.25 128.62,25.25 128.16,25.75 SV1.22
ADDRESS14
  Top 0.305: SV1.19 126.88,27 130.98,27 U6.48
  Bottom 0.305: U6.48 131.24,26.76 131,27 126.87,27 SV1.19
ADDRESS15
  Top 0.305: U6.1 131.28,8.22 130.38,9.25 126.84,9.25 SV1.33
  Bottom 0.305: SV1.33 125.6,10.46 126.81,9.25 130.31,9.25 131.25,8.31 131.25,7.33 U6.1
ADDRESS16
  Top 0.305: U6.2 131.78,6.28 131.44,5.81 130.75,5.81 128.56,7.94 128.59,7.94 SV1.36
  Bottom 0.305: SV1.36 128.55,7.95 130.75,5.81 131.44,5.81 131.78,6.28 131.78,6.43 U6.2
ADDRESS17
  Top 0.305: U6.3 132.28,8.72 130.5,10.5 128.15,10.5 SV1.34
  Bottom 0.305: SV1.34 130.51,10.49 132.25,8.75 132.28,8.27 U6.3
ADDRESS18
  Top 0.305: U6.4 132.78,5.85 132,5.06 130.31,5.06 128.81,6.62 126.93,6.62 SV1.35
  Bottom 0.305: SV1.35 125.6,7.9 126.94,6.62 128.81,6.62 130.31,5.06 132,5.06 132.78,5.84 132.78,6.43 U6.4
ADDRESS19
  Top 0.305: U6.5 133.28,9.53 131.19,11.75 126.88,11.75 SV1.31
  Bottom 0.305: SV1.31 125.66,13.03 126.88,11.75 131.19,11.75 133.28,9.53 133.28,8.21 U6.5
BTN0  (via drill 0.6)
  Top 0.305: R17.1 25.16,42.12 R20.2 25.31,41.97 25.31,40.56 27.88,38 115.19,38 115.69,38.5 v115.75,38.5
  Bottom 0.305: SV1.6 128.11,46.05 126.88,44.81 122.06,44.81 v115.75,38.5
BTN1  (via drill 0.6)
  Top 0.305: v118.44,37.69 118,37.25 23.94,37.25 22.2,38.99 R19.2 R18.1
  Bottom 0.305: SV1.8 126.88,42.25 123,42.25 v118.44,37.69
BTN2  (via drill 0.6)
  Top 0.305: R23.1 46.68,42.06 R26.2 46.62,41.97 46.62,41.12 48.38,39.38 112.88,39.38 114,40.5 v114,40.56
  Bottom 0.305: SV1.1 124.57,51.13 v114,40.56
BTN3  (via drill 0.6)
  Top 0.305: v115.56,40.31 113.94,38.69 44.81,38.69 43.56,40 43.56,40.52 R25.2 43.55,45.07 R24.1
  Bottom 0.305: SV1.3 123.84,48.59 v115.56,40.31
CK_CLK  (via drill 0.6)
  Top 0.305: SV3.4 111.33,35.21 112.19,36.06 121.19,36.06 v121.56,36.38
  Bottom 0.305: v121.56,36.38 122.44,37.12 131.12,37.12 137.5,43.5 143.38,43.5 144.69,44.81 147.23,44.81 SV2.6
CK_DAT
  Top 0.305: SV3.3 108.79,32.33 110.06,31.06 118.44,31.06 124.56,37.12 131.12,37.12 137.5,43.5 SV2.7
CS_B
  Top 0.305: U6.7 134.28,6.28 132.06,4.12 129.5,4.12 128.44,5.12 128.24,5.31 SV1.38
CS_T
  Bottom 0.305: SV2.37 144.62,4.12 141.75,4.12 139.78,6.09 U5.7
DATA0
  Top 0.305: U6.17 139.28,5.84 142.25,2.88 145.8,2.88 SV2.39
  Bottom 0.305: SV2.39 142.25,2.87 139.28,5.84 139.28,7.21 U6.17
DATA1
  Top 0.305: U6.16 138.78,9.41 142.44,13.06 145.89,13.06 SV2.31
  Bottom 0.305: SV2.31 142.53,13.09 138.78,9.41 138.78,8.2 U6.16
DATA2
  Top 0.305: U6.15 138.34,4.59 142,1.19 146.91,1.19 SV2.40
  Bottom 0.305: SV2.40 148.46,2.84 146.88,1.19 142,1.19 138.31,4.62 138.31,6.21 U6.15
DATA3
  Top 0.305: SV2.28 148.46,18.09 147.25,16.88 144.44,16.88 137.78,10.25 137.78,8.33 U6.14
  Bottom 0.305: U6.14 137.78,10.25 144.44,16.88 147.23,16.88 SV2.28
DATA4
  Top 0.305: U6.11 136.28,10.22 129.69,16.81 126.84,16.81 SV1.27
  Bottom 0.305: U6.11 136.28,10.22 129.69,16.81 126.84,16.81 SV1.27
DATA5
  Top 0.305: U6.10 135.78,4.35 133.12,1.69 126.66,1.69 SV1.39
  Bottom 0.305: SV1.39 125.6,2.83 126.69,1.69 133.12,1.69 135.78,4.34 135.78,6.33 U6.10
DATA6
  Top 0.305: U6.9 135.28,9.65 131.94,13 128.17,13 SV1.32
  Bottom 0.305: SV1.32 131.91,13.03 135.28,9.66 135.28,8.3 U6.9
DATA7
  Top 0.305: U6.8 134.78,5.1 132.5,2.81 128.39,2.88 SV1.40
  Bottom 0.305: SV1.40 132.5,2.81 134.78,5.09 134.78,6.27 U6.8
DATA8
  Top 0.305: SV1.16 130.34,33.35 134.81,28.88 134.78,27.61 U6.41
  Bottom 0.305: U6.41 134.78,28.9 130.38,33.31 128.18,33.31 SV1.16
DATA9
  Top 0.305: U6.40 135.28,24.72 129.94,19.38 126.88,19.38 SV1.25
  Bottom 0.305: U6.40 135.28,24.72 129.94,19.38 126.89,19.38 SV1.25
DATA10
  Top 0.305: SV1.13 125.6,35.83 126.81,34.62 130.75,34.62 135.81,29.56 135.78,27.61 U6.39
  Bottom 0.305: U6.39 135.78,29.59 130.75,34.62 126.87,34.62 SV1.13
DATA11
  Top 0.305: U6.38 136.28,23.47 130.94,18.12 128.28,18.12 SV1.28
  Bottom 0.305: U6.38 136.28,23.47 130.94,18.12 128.47,18.12 SV1.28
DATA12
  Top 0.305: U6.35 137.78,23.47 143.12,18.12 145.91,18.12 SV2.27
  Bottom 0.305: U6.35 137.78,23.47 143.12,18.12 145.75,18.12 SV2.27
DATA13
  Top 0.305: U6.34 138.28,30.41 142.47,34.59 147.17,34.59 SV2.14
  Bottom 0.305: U6.34 138.28,30.41 142.47,34.59 147.17,34.59 SV2.14
DATA14
  Top 0.305: U6.33 138.78,23.78 143.12,19.44 147.25,19.44 SV2.26
  Bottom 0.305: U6.33 138.78,23.78 143.12,19.44 147.25,19.44 SV2.26
DATA15
  Top 0.305: U6.32 139.28,29.66 142.94,33.31 145.76,33.31 SV2.15
  Bottom 0.305: U6.32 139.28,29.66 142.94,33.31 145.89,33.31 SV2.15
GND  (via drill 0.6)
  Top 0.254: 137.44,5.62 arc7 137.31,6.31 arc-9 U6.13 | U4.3 14.09,52.16 | U2.3 46.56,51.94 47.06,51.44 50.12,51.44 v51.19,52.5
  Top 0.305: C11.2 135.9,31.29 136.78,30.4 U6.37 136.78,20.16 v135.56,18.94 | U6.13 137.28,14.66 v139,16.38 | 14.09,52.16 arc90 14.62,51.62 | U1.3 22.93,52.13 arc90 23.38,51.69 | U3.3 33.57,52.3 arc90 34.25,51.62
  Top 0.406: C14.2 137.56,2.66 | U3.8 32.28,55.65 32.12,55.5
  Top 0.61: 137.56,2.66 137.44,5.62
  Top 1.016: C11.2 135.93,32.02 C10.2
  Bottom 0.305: v135.56,18.94 133.56,16.94 133.56,15.88 136.78,12.65 U5.13 136.78,4.03 136.19,3.44 136.19,2.45 C13.2 | v139,16.38 139.81,17.19 139.81,19.5 137.28,22.03 U5.37 137.28,31.96 C12.2
  Bottom 0.813: C9.2 137.57,34.5
  Bottom 1.016: v139,16.38 v135.56,18.94 | 137.57,34.5 C12.2
  other vias: 131.5,17 142.56,16.94 139.69,34.25 45.25,43.5 65.19,51.81 65.25,50.12 58.44,53.44 29.69,52.62 25.44,52.62 17.62,52.56 132.06,41.12 139.5,45.56 133.38,34.75 23.81,43.38 22.25,50.06 10.5,65.38 37.25,58.62 150.5,13.75 139.56,71.38 17.12,55.62 28.75,58.56 39.56,52.44 28.5,39.19 25.56,38.5 28.12,36.06 50.81,40.69 42.31,39.5 46.69,36.19 117.69,38.88 114.12,44.94 114.19,47.06 117.38,47.44 119.25,48.69 120,51.19 111.44,41.25 122,1.06 94.69,1.06
  pour Bottom: 0,0 0,84.44 0.06,84.5 152.38,84.5 152.38,0.12 152.44,0.06 0.56,0.06 0.25,-0.25
  pour Top: 0.25,0.12 90,0.06 152.44,0 152.44,84.5 0.06,84.44
J_CLK0
  Top 0.254: U1.7 22.27,55.23 22.94,54.56 59.38,54.56 64.56,49.25 116.88,49.25 120.08,46.05 SV1.5
J_CLK1
  Top 0.254: U4.7 13.43,55.33 14.75,54 55.94,54 61.69,48.06 115.31,48.06 120.05,43.51 SV1.7
J_CLK2
  Top 0.254: U3.7 32.91,55.77 33.44,55.25 59.62,55.25 63.94,50.94 117.25,50.94 118.38,49.81 126.94,49.81 128.14,48.61 SV1.4
J_CLK3
  Top 0.254: U2.7 45.91,56.16 46.25,55.81 60.06,55.81 63.25,52.62 127.62,52.62 128.14,52.11 SV1.2
J_MCLK
  Top 0.305: R14.1 60.23,45.94 115.88,45.94 120.84,40.97 SV1.9
J_MCLK_R
  Top 0.254: R14.2 53.59,50.81 47.06,50.81 45.91,52.03 45.91,52.09 | U2.2 45.91,52.09 | 45.91,52.09 44.62,50.75 33.88,50.75 32.91,52.04 | U3.2 32.91,52.04 | 32.91,52.04 32,50.81 23.44,50.88 22.25,51.75 22.25,52.82 U1.2 22.27,51.77 21.31,50.94 14.25,50.94 13.44,52.06 13.44,52.83 U4.2
LB_B
  Top 0.305: U6.42 134.28,25.03 129.88,20.62 128.17,20.62 SV1.26
LB_T
  Bottom 0.305: U5.42 139.78,24.15 143.31,20.62 145.9,20.62 SV2.25
N$1
  Top 0.406: C1.1 135.6,63.34 U7.1
N$2
  Top 0.406: U7.3 138.15,66.08 137.44,65.38 137.44,63.46 C1.2
N$3
  Top 0.406: U7.4 139.41,63.49 C2.1
N$4
  Top 0.406: U7.5 140.69,65.88 141.19,65.38 141.19,63.37 C2.2
N$5
  Top 0.406: C3.1 133.35,69.03 134.25,70.12 136.5,70.12 136.88,69.69 U7.2
N$6
  Top 0.406: C4.1 142.91,64.59 142.06,65.44 142.06,68.2 U7.6
N$8
  Top 0.406: X1.2 118.03,71.41 121.25,68.19 129.31,68.19 133.25,72.12 138.5,72.12 139.44,73.06 139.44,74.43 U7.13
N$9
  Top 0.406: U7.7 143.22,69.28 142,70.12 137.75,70.12 136.88,71 133.44,71 129.12,66.69 119.96,66.69 X1.3
N$11  (via drill 0.6)
  Top 0.254: v50,49.31 50,48.75 R22.1
  Top 0.305: R23.2 48.56,45.2 R22.1
  Bottom 0.254: X3.4 49.94,68.72 v50,49.31
N$12
  Top 0.305: X2.1 12.67,68.39 R4.2 R3.1
N$13
  Top 0.305: R4.1 R7.2 15.29,57.73 U4.5
N$14
  Top 0.305: R5.1 R6.2 25.37,58.96 U1.5
N$15
  Top 0.305: X2.2 19.09,68.29 R2.1 R5.2
N$16  (via drill 0.6)
  Top 0.305: R24.2 41.81,47.19 R21.1 41.94,48.75 v42.5,49.44
  Bottom 0.254: X3.6 42.44,63.83 v42.5,49.44
N$17
  Top 0.305: X3.1 35.34,69.43 R9.1 R10.2
N$18
  Top 0.305: U3.5 34.21,58.85 R10.1 R13.2
N$19
  Top 0.305: U2.5 47.2,59.3 46.56,60.06 43.95,60.06 R12.2 R11.1
N$20
  Top 0.305: X3.2 40.84,68.3 R11.2 R8.1
N$21  (via drill 0.6)
  Top 0.254: v27.25,49 27.25,49.07 R16.1
  Top 0.305: R17.2 27.25,44.41 R16.1
  Bottom 0.254: X2.4 27.19,67.67 v27.25,49
N$22  (via drill 0.6)
  Top 0.254: v19.94,48.69 19.94,47.33 R15.1
  Top 0.305: R18.2 20.3,47.18 R15.1
  Bottom 0.254: X2.6 22.47,66.47 21,65 21,49.75 v19.94,48.69
N$27  (via drill 0.6)
  Top 0.406: R1.1 115.56,68.25 v115.75,68.44
  Bottom 0.406: v115.75,68.44 116.62,69.3 X1.7
N$28  (via drill 0.6)
  Top 0.406: U7.14 138.12,74.47 138.12,76 v137.62,76.62 | X1.4 112.5,68.31 R1.2
  Bottom 0.406: v137.62,76.62 137.31,76.31 113.75,76.31 112.44,75 112.44,71.47 X1.4
OE_B
  Top 0.305: SV1.15 125.65,33.35 126.88,32.12 129.75,32.12 133.25,28.62 133.28,28.07 U6.44
OE_T
  Bottom 0.305: U5.44 140.78,29.91 142.94,32.06 147.18,32.06 SV2.16
RST
  Top 0.305: SV2.5 142.45,46.05 128.81,59.69 91.62,59.69 86.19,65.12 86.19,68.62 SV4.4
RW_B
  Top 0.305: SV2.38 147.19,4.12 141.75,4.12 139.78,6.09 139.78,6.49 U6.18
RW_T
  Bottom 0.305: SV1.37 125.6,5.4 126.88,4.12 132.06,4.12 134.28,6.28 134.28,6.43 U5.18
RXD0
  Top 0.406: SV2.1 145.92,51.74 146.88,52.75 146.81,69.25 145.69,70.5 143.75,70.5 140.75,72.31 140.75,74.39 U7.12
TXD0
  Top 0.406: U7.10 143.22,73.28 144.38,72.19 147.06,72.19 148.69,70.56 148.69,51.35 SV2.2
UB_B
  Top 0.305: U6.43 133.78,25.53 130.19,21.94 126.86,21.94 SV1.23
UB_T
  Bottom 0.305: U5.43 140.28,25.03 143.44,21.88 147.15,21.88 SV2.24
WF_RXD
  Top 0.305: SV4.1 96.23,71.27 104.56,62.94 130.19,62.94 143.19,49.88 147.12,49.88 SV2.4
WF_TXD
  Top 0.305: SV2.3 145.39,48.56 141.94,48.62 129.25,61.38 92.19,61.38 87.56,65.94 87.62,69.38 87,70 82.43,70 SV4.8

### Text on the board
Top: GLB | WiFi | CoCo3FPGA Analog Board | +3V3 | RTC | +5V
